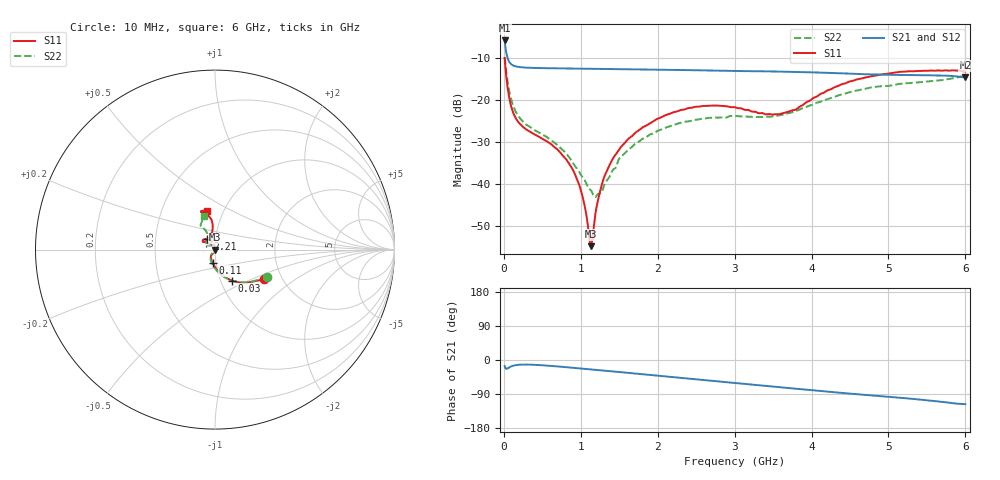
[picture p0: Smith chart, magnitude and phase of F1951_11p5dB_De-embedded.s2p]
! Integrated Device Technology
! Corporate Headquarters
! 6024 Silver Creek Valley Road
! San Jose, CA 95138  USA
! Phone:  1-408-284-8200
! Toll Free:  1-800-223-1366
! Webpage:  http://www.idt.com/
! Timing and RF Division
! 515 Groton Road, Suite 102
! Westford, MA 01886-6024
! Device:  F1951
! Description: 6-bit 0.5 dB Digital Step Attenuator
! Frequency:  100.0 -  4000.00 MHz
! Package:  4x4 mm Thin QFN Plastic Package: 24 pin
! Ports:  2 RF, 6 DC
!  Pin  1  = NC
!  Pin  2  = RF1  =  Port 1
!  Pin  3  = GND
!  Pin  4  = NC
!  Pin  5  = Serial Data Out (SDO)
!  Pin  6  = NC
!  Pin  7  = Reset Bar ( RSTb)
!  Pin  8  = Clock (CLK)
!  Pin  9  = Chip Select Bar (CSb)
!  Pin 10  = NC
!  Pin 11  = Serial Data In (SDI)
!  Pin 12  = NC
!  Pin 13  = NC
!  Pin 14  = VDD
!  Pin 15  = NC
!  Pin 16  = GND
!  Pin 17  = RF2  =  Port 2
!  Pin 18  = NC
!  Pin 19  = GND
!  Pin 20  = GND
!  Pin 21  = GND
!  Pin 22  = GND
!  Pin 23  = GND
!  Pin 24  = GND
! State:  23
! Atten State:  11.5 dB
! Voltage:  +3.30 Volts
! Current:  0.486 mA
! Data:  The device was measured on a F195X evaluation board which has
!  individual transmission lines to the RF pins.  Data was collected
!  de-embedded using a Automatic Fixture Removal [AFR] (Keysight Technologies).
!  The reference plane is the edge of the package pin.
! Misc:  Lot Code  1225BCA
!  Action Tracker AT0399
! Date Measured:  2018-09-13
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# GHz S dB R 50
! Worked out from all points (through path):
!   600 points, 10 MHz to 6 GHz, reference 50 ohm
!   highest |S21| = -5.74 dB at 10 MHz (marker M1); lowest = -14.6 dB at 6 GHz (marker M2)
!   group delay of S21, straight-line fit = 50.9 ps
!   lowest |S11| = -54.8 dB at 1.13 GHz (marker M3), VSWR 1.00, Z = 49.8 + j0.0159 ohm
!   |S11| at or under -10 dB: 10.23 MHz to end of sweep
!   |S22| runs from -43.1 to -9.7 dB; largest |S21 - S12| = 0.00042
!   S11 on the Smith chart (normalised r, x): 10 MHz: 1.61, -0.60; 30 MHz: 1.13, -0.41; 110 MHz: 0.97, -0.15; 2.21 GHz: 0.91, +0.11; 6 GHz: 0.84, +0.38
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0.01  -9.95 -31.5  -5.74 -16.0  -5.75 -16.0  -9.69 -27.2
0.03  -14.06 -61.5  -8.45 -23.3  -8.45 -23.4  -13.03 -54.5
0.07  -19.40 -86.6  -10.84 -19.6  -10.85 -19.7  -17.80 -81.0
0.11  -22.39 -99.2  -11.60 -15.8  -11.60 -15.8  -20.69 -94.9
0.26  -26.53 -119.2  -12.19 -12.0  -12.20 -11.9  -25.38 -117.9
0.8  -33.88 -117.4  -12.42 -18.8  -12.42 -18.7  -32.52 -127.2
0.91  -37.09 -114.1  -12.46 -20.7  -12.46 -20.7  -35.29 -128.2
1.01  -42.06 -114.6  -12.48 -22.5  -12.48 -22.5  -38.04 -132.2
1.13  -54.84 174.9  -12.50 -24.6  -12.50 -24.6  -41.51 -154.2
1.15  -53.30 137.9  -12.50 -25.0  -12.50 -25.0  -42.12 -160.5
1.19  -47.19 108.7  -12.51 -25.7  -12.51 -25.7  -43.14 -177.6
1.27  -40.39 97.3  -12.52 -27.3  -12.52 -27.2  -42.04 152.6
1.41  -34.16 98.2  -12.55 -29.9  -12.55 -29.9  -36.88 127.7
1.62  -29.20 105.0  -12.59 -33.9  -12.60 -34.0  -31.82 121.4
2.01  -24.34 119.5  -12.70 -41.6  -12.71 -41.6  -27.21 129.4
2.21  -22.85 126.5  -12.77 -45.5  -12.77 -45.5  -25.89 134.8
3.01  -21.72 146.7  -13.02 -60.9  -13.03 -60.8  -23.72 149.1
3.58  -23.34 122.8  -13.17 -71.7  -13.17 -71.7  -23.60 130.4
4.01  -19.65 98.2  -13.35 -79.8  -13.35 -79.8  -21.09 117.2
4.49  -15.57 96.7  -13.66 -88.5  -13.66 -88.5  -18.14 116.9
5.01  -13.61 105.8  -13.95 -97.1  -13.95 -97.1  -16.58 120.8
6  -13.12 101.6  -14.57 -116.5  -14.57 -116.5  -14.14 108.7
